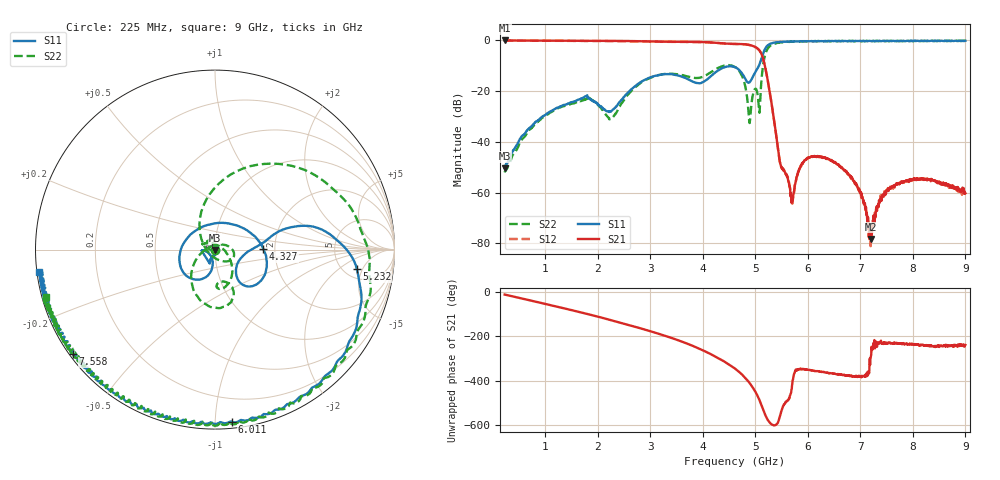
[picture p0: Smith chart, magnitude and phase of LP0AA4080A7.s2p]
!Agilent Technologies,E8358A,US41080443,A.07.50.56
!Agilent E8358A: A.07.50.56
!Date: Tuesday, January 09, 2018 21:38:31
!Correction: S11(Full 2 Port(1,2))
!S21(Full 2 Port(1,2))
!S12(Full 2 Port(1,2))
!S22(Full 2 Port(1,2))
!S2P File: Measurements: S11, S21, S12, S22:
# Hz S  dB  R 50
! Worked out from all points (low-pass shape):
!   1601 points, 225 MHz to 9 GHz, reference 50 ohm
!   highest |S21| = 0.00 dB at 236 MHz (marker M1); lowest = -78.3 dB at 7.201 GHz (marker M2)
!   |S21| within 3 dB of the highest: start of sweep to 5.032 GHz
!   lowest |S11| = -50.4 dB at 225 MHz (marker M3), VSWR 1.01, Z = 50.2 - j0.249 ohm
!   |S11| at or under -10 dB: start of sweep to 5.067 GHz
!   |S22| runs from -52.0 to -0.1 dB; largest |S21 - S12| = 0.0091
!   S11 on the Smith chart (normalised r, x): 225 MHz: 1.00, -0.00; 4.327 GHz: 1.74, +0.01; 5.232 GHz: 6.53, -3.88; 6.011 GHz: 0.04, -1.10; 7.558 GHz: 0.01, -0.33; 9 GHz: 0.01, -0.06
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2.25e8  -50.35 -54.9  -0.01 -12.3  -0.06 -12.3  -52.01 -122.3
2.359688e8  -49.67 -53.4  -0.00 -12.9  -0.06 -12.9  -51.53 -124.2
8.227969e8  -32.02 -88.6  -0.07 -44.8  -0.12 -44.7  -32.40 -175.3
1.689328e9  -22.81 -114.9  -0.15 -93.3  -0.20 -93.2  -23.82 110.1
2.254219e9  -27.91 -129.6  -0.17 -127.4  -0.23 -127.3  -30.96 58.4
3.153656e9  -13.67 -128.6  -0.44 171.5  -0.51 171.7  -13.67 -70.1
3.888562e9  -16.77 118.2  -0.57 108.7  -0.61 109.0  -14.77 -78.1
4.327312e9  -11.38 0.6  -1.05 57.3  -1.10 57.6  -10.53 -71.5
4.6125e9  -10.55 -42.2  -1.36 14.6  -1.40 14.9  -10.43 -103.7
4.766062e9  -13.61 -52.5  -1.45 -16.8  -1.50 -16.4  -14.98 -136.9
4.897688e9  -16.30 -17.2  -1.80 -52.8  -1.85 -52.5  -31.65 79.3
5.095125e9  -8.50 16.1  -4.45 -136.9  -4.53 -136.6  -22.43 152.3
5.232234e9  -1.96 -7.8  -15.31 145.1  -15.34 145.9  -3.32 39.1
5.468062e9  -0.58 -44.9  -47.93 160.4  -48.06 158.2  -0.82 -22.9
5.687438e9  -0.42 -64.3  -63.97 -80.8  -62.78 -80.5  -0.45 -48.3
6.011016e9  -0.31 -84.3  -46.31 8.8  -46.06 10.2  -0.26 -70.5
6.076828e9  -0.32 -87.8  -45.82 5.7  -45.69 6.1  -0.25 -74.3
6.822703e9  -0.24 -119.6  -53.55 -19.5  -53.94 -18.2  -0.32 -107.7
7.201125e9  -0.29 -133.1  -78.28 68.9  -79.72 44.2  -0.20 -121.9
7.541156e9  -0.22 -142.9  -58.93 130.5  -59.01 128.9  -0.30 -132.7
7.557609e9  -0.14 -143.6  -58.06 128.9  -58.54 132.3  -0.30 -132.3
9e9  -0.11 -172.8  -60.25 121.1  -60.26 120.7  -0.20 -164.2
